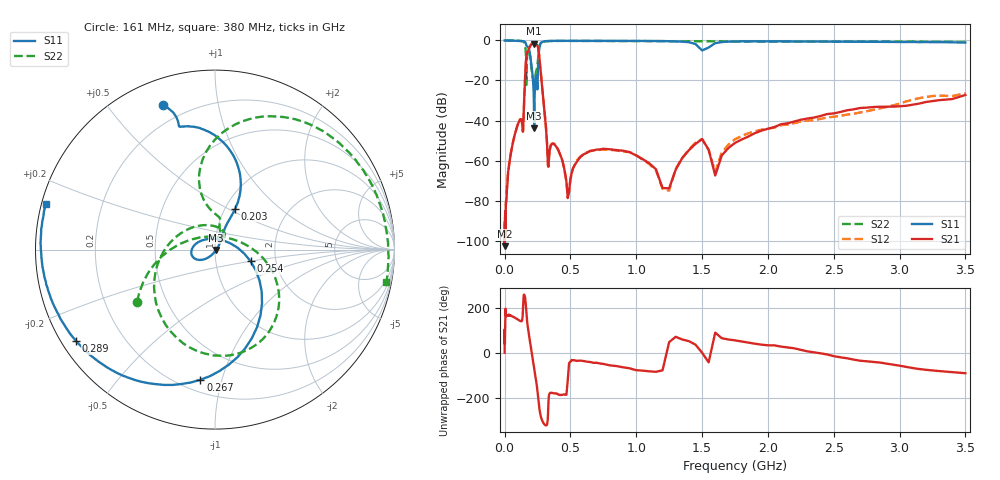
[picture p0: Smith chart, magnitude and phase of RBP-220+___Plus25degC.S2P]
! Mini-Circuits
! S2P DATA File Format
! Type: BAND PASS FILTER
! Model: RBP-220+
! All S Parameters are in dB deg format
! TEST CONDITIONS: INPUT POWER = 0 dBm @ Temperature = + 25 deg C
! 401 Frequency points
# MHz S DB R 50
!FREQ  MAG(S11)PHS(S11)MAG(S21)PHS(S21)MAG(S12)PHS(S12)MAG(S22)PHS(S22)
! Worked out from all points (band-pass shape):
!   401 points, 500 kHz to 3.5 GHz, reference 50 ohm
!   highest |S21| = -1.62 dB at 220 MHz (marker M1); lowest = -102.8 dB at 1 MHz (marker M2)
!   |S21| within 3 dB of the highest: 183.1 MHz to 257.5 MHz (74.38 MHz wide, 33.8 % of centre)
!   lowest |S11| = -43.9 dB at 225 MHz (marker M3), VSWR 1.01, Z = 50.6 - j0.243 ohm
!   |S11| at or under -10 dB: 199.6 MHz to 256.3 MHz (56.67 MHz wide, 24.9 % of centre)
!   |S22| runs from -22.2 to 0.0 dB; largest |S21 - S12| = 0.011
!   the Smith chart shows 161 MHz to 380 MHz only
!   S11 on the Smith chart (normalised r, x): 161 MHz: 0.12, +0.70; 203 MHz: 1.11, +0.54; 254 MHz: 1.48, -0.20; 267 MHz: 0.28, -0.86; 289 MHz: 0.04, -0.30; 380 MHz: 0.01, +0.13
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0.5  -0.02 179.9  -99.51 1.4  -90.18 -88.4  -0.01 -0.2
1  -0.03 179.7  -102.77 105.5  -98.99 7.3  -0.01 -0.3
2.5  -0.03 179.3  -90.98 40.9  -96.29 174.6  0.00 -0.7
10  -0.04 177.3  -81.09 166.7  -82.73 -166.5  -0.01 -3.1
42.5  -0.09 169.1  -58.67 164.6  -58.33 164.7  -0.01 -13.4
139  -0.34 132.8  -45.53 -176.9  -45.50 -176.1  -0.42 -70.5
161  -1.38 109.7  -12.23 -140.4  -12.16 -141.0  -5.63 -146.1
166.5  -2.60 106.1  -7.46 176.5  -7.41 176.0  -21.95 62.5
183  -3.89 90.4  -4.63 90.2  -4.67 90.0  -4.70 -95.5
203  -11.88 63.7  -1.99 13.5  -1.97 13.1  -13.42 155.4
220  -24.14 57.5  -1.62 -48.2  -1.62 -48.3  -19.96 56.7
225  -43.91 -22.1  -1.65 -66.0  -1.64 -66.0  -20.75 61.5
254  -13.63 -18.0  -3.44 171.5  -3.49 171.2  -9.03 103.8
267  -2.74 -96.4  -10.31 105.6  -10.34 107.0  -2.24 72.5
289  -0.67 -146.7  -25.57 57.8  -25.51 57.6  -0.68 34.8
330  -0.28 -177.7  -62.11 90.2  -62.35 89.7  -0.35 6.8
380  -0.20 164.8  -52.18 -178.3  -51.70 -177.9  -0.25 -10.8
480  -0.18 144.1  -78.76 -120.3  -77.90 -146.6  -0.22 -32.5
850  -0.19 92.0  -54.77 -57.3  -54.94 -60.0  -0.30 -84.6
1250  -0.39 34.3  -73.87 48.3  -75.02 59.8  -0.36 -131.5
2450  -0.56 -84.5  -36.76 -6.1  -38.49 -2.9  -0.48 99.8
3500  -1.04 143.5  -27.23 -88.9  -26.40 -97.3  -0.75 -11.0
